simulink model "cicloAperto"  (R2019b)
settings: Solver=FixedStepDiscrete  StartTime=0.0  StopTime=50  FixedStep=1  RelTol=1e-3

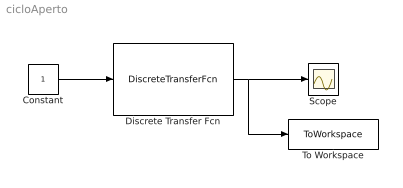
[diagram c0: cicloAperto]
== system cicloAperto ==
  Constant : Constant
  Discrete Transfer Fcn : DiscreteTransferFcn  Denominator=[1 -0.3 -0.4]
  Scope : Scope
  To Workspace : ToWorkspace  VariableName=y  SaveFormat=Timeseries  SampleTime=-1
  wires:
  Constant/1 -> Discrete Transfer Fcn/1
  Discrete Transfer Fcn/1 -> Scope/1, To Workspace/1
